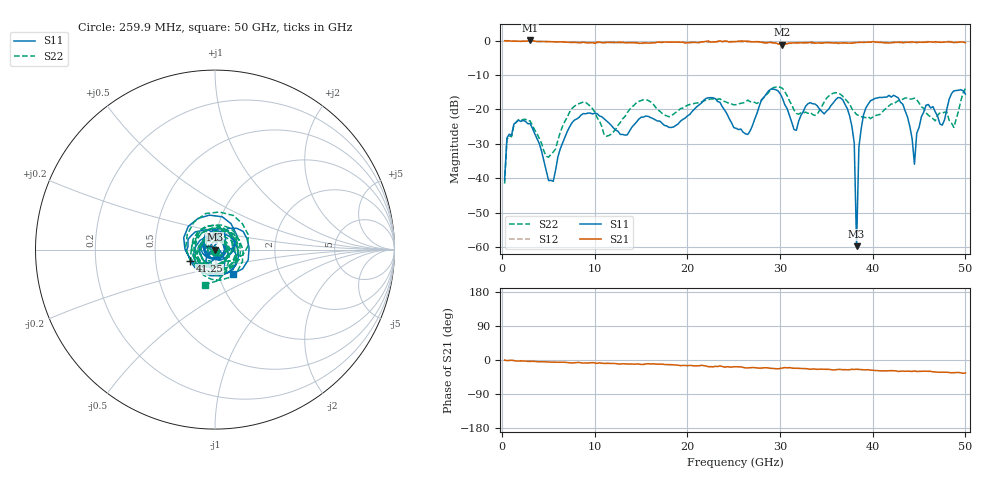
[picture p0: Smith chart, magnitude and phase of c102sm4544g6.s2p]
! 5/5/2022 10:44:04 AM
! D:\C102SM4544G6.S2P
! CHANNEL.1
! TR.MEASUREMENT
! CORRECTED.DATA
# GHZ S RI R 50.0
! FREQ.GHZ  S11RE  S11IM  S21RE  S21IM  S12RE  S12IM  S22RE  S22IM
!; PortSelection: Port_12
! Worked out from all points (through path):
!   200 points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, 259.9 MHz to 50 GHz, reference 50 ohm
!   highest |S21| = 0.07 dB at 3.009 GHz (marker M1); lowest = -1.1 dB at 30.25 GHz (marker M2)
!   group delay of S21, straight-line fit = 1.79 ps
!   lowest |S11| = -59.8 dB at 38.25 GHz (marker M3), VSWR 1.00, Z = 49.9 + j0.054 ohm
!   |S11| at or under -10 dB: start of sweep to end of sweep
!   |S22| runs from -41.6 to -13.3 dB; largest |S21 - S12| = 0.051
!   S11 on the Smith chart (normalised r, x): 259.9 MHz: 0.99, -0.02; 41.25 GHz: 0.75, -0.10; 50 GHz: 1.17, -0.33
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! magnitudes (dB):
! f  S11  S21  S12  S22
! 259.9 MHz  -40.5  0.0  0.0  -41.6
! 509.9 MHz  -28.3  0.0  0.0  -28.7
! 3.009 GHz  -24.1  0.1  0.0  -23.3
! 5.509 GHz  -40.9  -0.3  -0.3  -32.4
! 8.758 GHz  -21.2  -0.5  -0.5  -17.8
! 11.26 GHz  -23.3  -0.5  -0.5  -27.8
! 17.01 GHz  -23.4  -0.4  -0.3  -20.5
! 25.25 GHz  -25.5  -0.3  -0.3  -18.6
! 30.25 GHz  -16.7  -1.1  -1.0  -13.9
! 31.75 GHz  -26.1  -0.6  -0.7  -21.1
! 33.5 GHz  -18.3  -0.5  -0.8  -21.5
! 37.5 GHz  -21.9  -0.7  -0.7  -18.4
! 38 GHz  -29.7  -0.6  -0.5  -20.6
! 38.25 GHz  -59.8  -0.5  -0.5  -21.5
! 38.5 GHz  -31.0  -0.5  -0.4  -21.8
! 39 GHz  -21.6  -0.5  -0.4  -22.2
! 41.25 GHz  -16.4  -0.6  -0.5  -20.1
! 41.75 GHz  -15.9  -0.7  -0.6  -18.9
! 44.5 GHz  -35.9  -0.5  -0.5  -16.7
! 45.75 GHz  -18.8  -0.4  -0.3  -21.0
! 48.75 GHz  -14.6  -0.6  -0.4  -25.2
! 50 GHz  -15.5  -0.6  -0.4  -13.9
